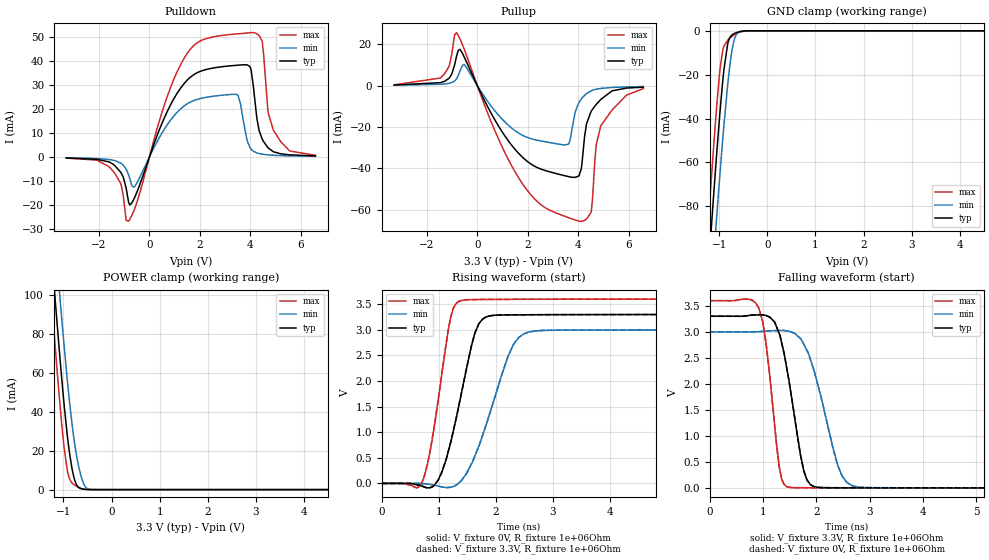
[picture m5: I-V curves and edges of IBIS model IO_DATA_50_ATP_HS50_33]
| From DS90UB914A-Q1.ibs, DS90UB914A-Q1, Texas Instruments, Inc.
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|   Model IO_DATA_50_ATP_HS50_33
[Model]  IO_DATA_50_ATP_HS50_33
Model_type   I/O
Polarity   Non-Inverting
Enable   Active-Low
Vinl =   0.8
Vinh =   2.0
Vmeas = 1.5000V
|   typ   min   max
|   (nom)   (fast)   (slow)
C_comp   1.107pF   0.7658pF   1.107pF
[Temperature Range]   25.0000   105.000   -40.0000
[Voltage Range]   3.3000V   3.0000V   3.6000V
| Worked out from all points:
|   slope of the pulldown table from 0 to 0.495 V, typ, clamps not added: 35.6 ohm
|   slope of the pullup table from 0 to 0.495 V, typ, clamps not added: 40.7 ohm
|   GND clamp passes 1 mA (typ) near -0.66 V on its own axis
|   POWER clamp passes 1 mA (typ) near -0.68 V on its own axis
|   falling waveform, V_fixture 3.3V, R_fixture 1e+06Ohm: 20-80 % time 315ps typ, 446ps min, 224ps max; typ from 3.3 V to 0 V
|   rising waveform, V_fixture 0V, R_fixture 1e+06Ohm: 20-80 % time 388ps typ, 532ps min, 287ps max; typ from 0 V to 3.3 V
|   rising waveform, V_fixture 3.3V, R_fixture 1e+06Ohm: 20-80 % time 388ps typ, 532ps min, 287ps max; typ from 0 V to 3.3 V
|   falling waveform, V_fixture 0V, R_fixture 1e+06Ohm: 20-80 % time 315ps typ, 446ps min, 224ps max; typ from 3.3 V to 0 V
[Pulldown]
|   Voltage   I(typ)   I(min)   I(max)
-3.3V     -399.6uA   -308.7uA   -443.4uA
-1.607V   -2.026mA   -1.041mA   -3.964mA
-1.142V   -6.328mA   -2.544mA   -10.99mA
-825mV    -18.93mA   -7.427mA   -26.76mA
-587.4mV  -16.86mA   -12.36mA   -21.6mA
1.472V    31.7mA     21.95mA    42.69mA
3.472V    38.2mA     26.04mA    51.26mA
4.125V    29.5mA     2.44mA     51.81mA
4.471V    7.592mA    1.207mA    48.3mA
4.699V    3.956mA    908.6uA    19.7mA
4.917V    2.215mA    736uA      11.25mA
6.59V     464.6uA    301.2uA    712.6uA
[GND Clamp]
|   Voltage   I(typ)   I(min)   I(max)
-3.3V     -802.8mA   -807.3mA   -804mA
-1.231V   -110.3mA   -138.1mA   -88.6mA
-1.201V   -100.9mA   -129mA     -79.02mA
-1.122V   -76.42mA   -105mA     -54.22mA
-1.073V   -61.58mA   -90.3mA    -39.6mA
-973.5mV  -33.94mA   -61.9mA    -15.45mA
-914.1mV  -19.88mA   -45.9mA    -7.711mA
-825mV    -5.965mA   -24.59mA   -4.279mA
-735.9mV  -1.901mA   -9.022mA   -2.567mA
-656.7mV  -953uA     -2.194mA   -1.419mA
-409.2mV  -17.01uA   -14.83uA   -33.8uA
6.59V     0A         0A         0A
[Pullup]
|   Voltage   I(typ)   I(min)   I(max)
-3.3V     325.6uA    225.9uA    413.3uA
-1.468V   1.449mA    673.1uA    3.717mA
-825mV    14.28mA    3.334mA    25.7mA
-508.2mV  13.56mA    10.03mA    17.3mA
1.749V    -34.12mA   -23.72mA   -46.68mA
3.61V     -43.98mA   -28.34mA   -63.84mA
4.125V    -40.3mA    -6.456mA   -65.63mA
4.333V    -18.49mA   -3.835mA   -64.59mA
4.511V    -12.58mA   -2.521mA   -61.34mA
4.719V    -9.085mA   -1.72mA    -28.63mA
4.897V    -6.702mA   -1.338mA   -19.52mA
6.59V     -717.4uA   -422.4uA   -1.422mA
[POWER Clamp]
|   Voltage   I(typ)   I(min)   I(max)
-3.3V     808mA      814.6mA    807.4mA
-1.31V    141.4mA    170.7mA    118.7mA
-1.241V   119.3mA    149.3mA    95.93mA
-1.211V   110mA      140.2mA    86.32mA
-1.132V   85.5mA     116.3mA    61.36mA
-1.092V   73.6mA     104.5mA    49.45mA
-1.003V   48.27mA    78.89mA    25.53mA
-924mV    28.79mA    57.57mA    10.55mA
-785.4mV  6.675mA    26.85mA    2.617mA
-646.8mV  602.8uA    8.134mA    725.3uA
-409.2mV  4.707uA    34.47uA    4.032uA
6.59V     0A         0A         0A
[Ramp]
R_load = 1e+06
|   typ   min   max
dV/dt_r   1.97991/3.87804e-10   1.79984/5.32329e-10   2.15993/2.86837e-10
dV/dt_f   1.97992/3.14723e-10   1.79985/4.46294e-10   2.15994/2.24027e-10
[Falling Waveform]
V_fixture = 3.3V
V_fixture_min = 3V
V_fixture_max = 3.6V
R_fixture = 1e+06Ohm
C_fixture = 0F
|   Time   V(typ)   V(min)   V(max)
0s        3.3V       3V         3.6V
920.6ps   3.328V     3.003V     3.46V
1.054ns   3.316V     3.015V     2.804V
1.305ns   2.962V     3.027V     396.8mV
1.446ns   2.297V     3.02V      21.45mV
1.701ns   640.7mV    2.872V     2.949mV
1.823ns   152.7mV    2.64V      2.478mV
2.401ns   2.445mV    430mV      1.225mV
2.671ns   1.782mV    40.85mV    1.029mV
10.05ns   113.2uV    182.4uV    88.99uV
[Rising Waveform]
V_fixture = 0V
V_fixture_min = 0V
V_fixture_max = 0V
R_fixture = 1e+06Ohm
C_fixture = 0F
|   Time   V(typ)   V(min)   V(max)
0s        8.697uV    46.8uV     2.249uV
711.8ps   -54.82mV   -2.462mV   37.54mV
988.1ps   64.26mV    -52.1mV    1.623V
1.211ns   816.3mV    -74.4mV    3.265V
1.391ns   1.732V     49.35mV    3.573V
1.629ns   2.929V     528.6mV    3.591V
1.765ns   3.207V     934.1mV    3.593V
2.209ns   3.292V     2.472V     3.596V
2.568ns   3.295V     2.954V     3.597V
10.05ns   3.3V       3V         3.6V
[Rising Waveform]
V_fixture = 3.3V
V_fixture_min = 3V
V_fixture_max = 3.6V
R_fixture = 1e+06Ohm
C_fixture = 0F
|   Time   V(typ)   V(min)   V(max)
0s        114.3uV    181.2uV    89.49uV
711.8ps   -54.6mV    -2.327mV   38.19mV
988.1ps   65.21mV    -51.81mV   1.624V
1.211ns   817.6mV    -73.57mV   3.266V
1.391ns   1.733V     50.55mV    3.573V
1.629ns   2.93V      530.2mV    3.591V
1.765ns   3.208V     935.8mV    3.593V
2.209ns   3.292V     2.474V     3.596V
2.568ns   3.295V     2.954V     3.597V
10.05ns   3.3V       3V         3.6V
[Falling Waveform]
|Gnd
V_fixture = 0V
V_fixture_min = 0V
V_fixture_max = 0V
R_fixture = 1e+06Ohm
C_fixture = 0F
|   Time   V(typ)   V(min)   V(max)
0s        3.3V       3V         3.6V
920.6ps   3.328V     3.003V     3.459V
1.054ns   3.316V     3.015V     2.804V
1.305ns   2.961V     3.027V     396.1mV
1.446ns   2.296V     3.02V      21.25mV
1.701ns   639.7mV    2.872V     2.824mV
1.823ns   152.2mV    2.64V      2.36mV
2.401ns   2.29mV     428.9mV    1.126mV
2.671ns   1.642mV    40.47mV    932.1uV
10.05ns   7.595uV    48.03uV    1.753uV
